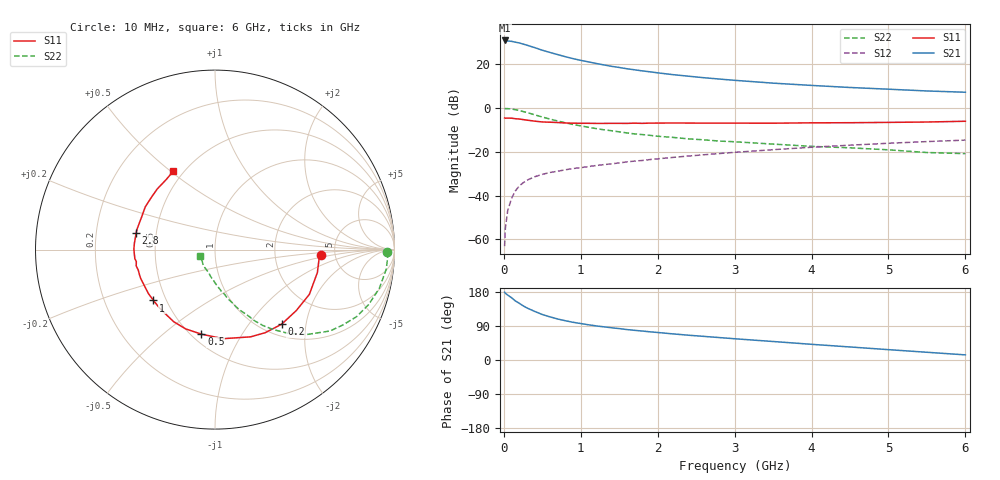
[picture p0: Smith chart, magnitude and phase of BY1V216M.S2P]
! SIEMENS Small Signal Semiconductors
! BFY420
! Si NPN RF SIEGET Grounded Emitter Transistor in MICRO-X
! VCE = 1.25 V  IC = 16 mA
! Common Emitter S-Parameters:  October  1996
# GHz  S  MA  R  50
!  f  S11  S21  S12  S22
! GHz  MAG  ANG  MAG  ANG  MAG  ANG  MAG  ANG
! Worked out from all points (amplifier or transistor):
!   36 points, 10 MHz to 6 GHz, reference 50 ohm
!   highest |S21| = 30.8 dB at 10 MHz (marker M1)
!   |S21| within 3 dB of that: start of sweep to 376.1 MHz
!   unconditionally stable (mu >= 1): 2.026 GHz to end of sweep
!   at 250 MHz: K = 0.26, MSG = 31.7 dB, |S12| = -34.2 dB
!   at 1.4 GHz: K = 0.88, MSG = 22.2 dB, |S12| = -25.5 dB
!   at 6 GHz: K = 1.09, MAG = 9.1 dB, |S12| = -14.7 dB
!   S11 on the Smith chart (normalised r, x): 10 MHz: 3.83, -0.35; 200 MHz: 1.21, -1.46; 500 MHz: 0.56, -0.68; 1 GHz: 0.43, -0.30; 2.8 GHz: 0.38, +0.09; 6 GHz: 0.44, +0.51
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0.01  0.589 -2.9  34.51 179.0  0.0007 105.7  0.9598 -0.9
0.02  0.5821 -5.3  34.29 176.1  0.0018 88.9  0.9631 -2.3
0.05  0.5846 -12.6  33.55 171.4  0.0045 87.6  0.9604 -6.5
0.1  0.5819 -25.4  32.93 164.3  0.0086 81.2  0.9408 -13.3
0.15  0.5661 -36.9  31.57 155.9  0.0128 73.8  0.9092 -19.7
0.2  0.5573 -48.3  30.26 149.8  0.0165 72.5  0.8733 -25.3
0.25  0.541 -58.8  28.59 143.1  0.0195 66.4  0.8261 -30.6
0.3  0.525 -67.8  26.92 137.4  0.0223 64.9  0.7849 -35.3
0.4  0.4984 -84.8  23.7 128.3  0.0268 59.4  0.6953 -42.9
0.5  0.4773 -99.1  20.66 120.0  0.0304 56.5  0.6187 -48.9
0.6  0.4711 -110.3  18.38 113.8  0.0336 54.5  0.5551 -53.6
0.7  0.463 -119.8  16.42 108.2  0.0359 53.9  0.5023 -57.6
0.8  0.4518 -128.2  14.7 103.6  0.0387 52.3  0.4556 -60.8
1  0.4448 -140.4  12.14 96.2  0.0433 52.2  0.3878 -65.4
1.1  0.4445 -146.4  11.19 92.9  0.0458 52.4  0.3612 -68.0
1.6  0.4426 -165.1  7.805 80.3  0.0586 52.0  0.2684 -76.7
2.2  0.4518 179.6  5.727 68.9  0.0742 50.7  0.2119 -84.9
2.8  0.4494 167.8  4.547 59.2  0.0909 48.2  0.1748 -92.2
3.5  0.4473 156.1  3.665 48.8  0.1112 44.2  0.1492 -100.1
4.5  0.4585 140.8  2.918 34.4  0.1409 36.1  0.1226 -112.8
5.5  0.4758 124.8  2.431 20.4  0.1701 27.0  0.0958 -138.6
6  0.495 117.9  2.272 13.5  0.1838 22.0  0.0904 -156.9
